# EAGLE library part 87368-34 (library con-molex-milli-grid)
RECEPTACAL
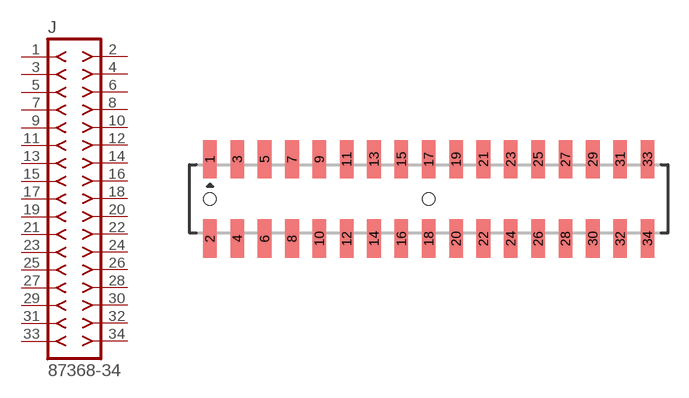
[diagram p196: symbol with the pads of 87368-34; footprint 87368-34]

Designator prefix J

## 87368-34  [87368-34]
1  1  pas
2  2  pas
3  3  pas
4  4  pas
5  5  pas
6  6  pas
7  7  pas
8  8  pas
9  9  pas
10  10  pas
11  11  pas
12  12  pas
13  13  pas
14  14  pas
15  15  pas
16  16  pas
17  17  pas
18  18  pas
19  19  pas
20  20  pas
21  21  pas
22  22  pas
23  23  pas
24  24  pas
25  25  pas
26  26  pas
27  27  pas
28  28  pas
29  29  pas
30  30  pas
31  31  pas
32  32  pas
33  33  pas
34  34  pas

## Footprint 87368-34 (pad centres in mm)
RECEPTACAL SMD Dual Row, Side Entry
smd 1 x 2.8: 1 -16,2.9; 2 -16,-2.9; 3 -14,2.9; 4 -14,-2.9; 5 -12,2.9; 6 -12,-2.9; 7 -10,2.9; 8 -10,-2.9; 9 -8,2.9; 10 -8,-2.9; 11 -6,2.9; 12 -6,-2.9; 13 -4,2.9; 14 -4,-2.9; 15 -2,2.9; 16 -2,-2.9; 17 0,2.9; 18 0,-2.9; 19 2,2.9; 20 2,-2.9; 21 4,2.9; 22 4,-2.9; 23 6,2.9; 24 6,-2.9; 25 8,2.9; 26 8,-2.9; 27 10,2.9; 28 10,-2.9; 29 12,2.9; 30 12,-2.9; 31 14,2.9; 32 14,-2.9; 33 16,2.9; 34 16,-2.9
hole 0.914 at -16,0
hole 0.914 at 0,0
